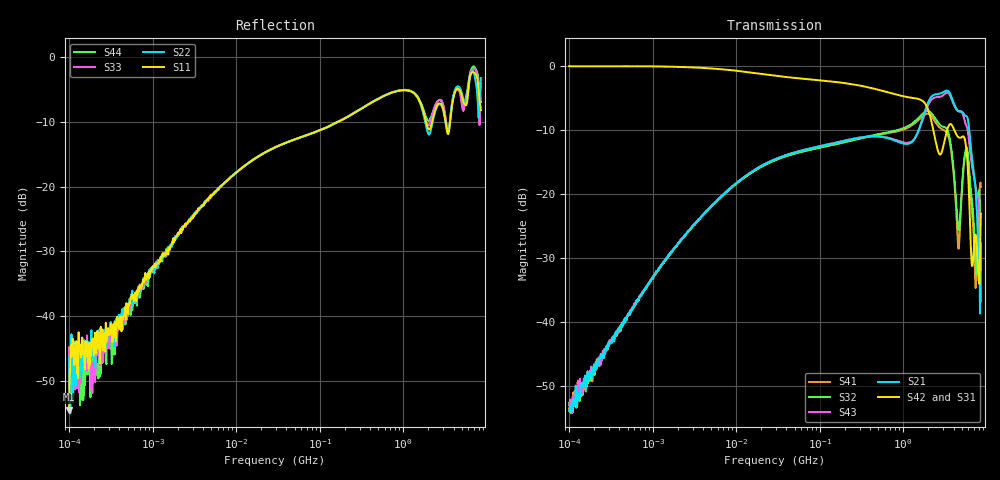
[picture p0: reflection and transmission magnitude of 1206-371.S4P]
!Agilent Technologies,E5071C,MY46110495,A.10.06
!Date: Tue Jun 06 11:07:04 2017
!Data & Calibration Information:
!Freq	S11:SOLT4(ON)	S12:SOLT4(ON)	S13:SOLT4(ON)	S14:SOLT4(ON)
!	S21:SOLT4(ON)	S22:SOLT4(ON)	S23:SOLT4(ON)	S24:SOLT4(ON)
!	S31:SOLT4(ON)	S32:SOLT4(ON)	S33:SOLT4(ON)	S34:SOLT4(ON)
!	S41:SOLT4(ON)	S42:SOLT4(ON)	S43:SOLT4(ON)	S44:SOLT4(ON)
!PortZ  Port1:50+j0  Port2:50+j0  Port3:50+j0  Port4:50+j0
!Above PortZ is port z conversion or system Z0 setting when saving the data.
!When reading, reference impedance value at option line is always used.
# Hz S dB R 50
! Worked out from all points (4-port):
!   801 points, 100 kHz to 8.5 GHz, reference 50 ohm
!   strongest paths, dB at 100 kHz, 1.721 MHz, 29.51 MHz, 502.3 MHz, 8.5 GHz:
!     S42: 0.0, -0.1, -1.5, -3.7, -23.1
!     S31: -0.1, -0.1, -1.5, -3.7, -27.3
!     S21: -53.9, -29.0, -14.6, -11.0, -27.8
!     S43: -53.1, -28.8, -14.6, -11.0, -27.8
!     S32: -52.7, -29.0, -14.7, -10.7, -28.0
!     S41: -53.5, -28.9, -14.7, -10.8, -18.9
!   lowest |S11| = -54.4 dB at 100 kHz (marker M1), VSWR 1.00, Z = 50.2 + j0.105 ohm
!   |S11| at or under -10 dB: start of sweep to 166.2 MHz; 1.867 GHz to 2.221 GHz (354.1 MHz wide, 17.3 % of centre); 3.211 GHz to 3.64 GHz (429 MHz wide, 12.5 % of centre)
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100000  -54.36 33.3  -55.71 82.1  -0.05 0.1  -53.83 -91.9
        -53.93 79.1  -46.27 7.1  -54.93 -84.9  -0.06 0.1
        -0.06 0.1  -52.70 -91.7  -44.76 96.1  -53.06 92.1
        -53.53 -99.3  -0.04 -0.1  -53.09 97.8  -47.70 63.1
9370604  -18.19 49.6  -18.64 47.9  -0.71 -5.9  -18.79 -132.7
         -18.66 48.0  -18.13 49.1  -18.74 -132.7  -0.71 -5.8
         -0.72 -5.8  -18.78 -132.9  -18.18 49.4  -18.64 47.9
         -18.70 -132.8  -0.70 -5.8  -18.64 48.0  -18.11 49.7
1.14275e9  -5.21 38.5  -12.17 22.4  -4.87 -34.1  -9.64 133.1
           -12.19 22.4  -5.18 37.2  -9.37 131.9  -4.91 -33.1
           -4.88 -34.1  -9.39 132.1  -5.21 36.7  -12.05 19.0
           -9.63 133.2  -4.90 -33.1  -12.03 19.1  -5.13 39.1
2.337209e9  -8.82 103.7  -4.51 21.8  -10.33 -74.6  -8.46 57.1
            -4.51 21.9  -9.07 106.2  -7.90 55.2  -10.59 -71.9
            -10.34 -74.6  -7.92 55.3  -8.06 102.9  -5.01 17.9
            -8.46 57.1  -10.59 -71.9  -5.00 17.8  -7.93 98.7
4.31778e9  -5.05 -131.3  -6.68 -22.4  -10.71 -78.4  -22.87 -33.2
           -6.68 -22.3  -4.71 -130.1  -21.40 -30.7  -10.71 -73.2
           -10.72 -78.2  -21.44 -30.7  -5.19 -136.8  -6.79 -27.9
           -22.79 -33.2  -10.70 -73.2  -6.79 -27.9  -4.95 -129.2
6.738951e9  -2.37 14.7  -14.90 -70.5  -31.50 -173.4  -23.45 -39.5
            -14.87 -70.5  -2.24 10.4  -21.77 -44.2  -31.34 -123.3
            -31.48 -172.9  -21.74 -43.8  -2.10 13.8  -16.07 -66.2
            -23.45 -39.3  -31.28 -122.9  -16.04 -65.9  -1.58 15.1
8.5e9  -8.23 103.2  -27.76 52.9  -27.28 86.5  -18.94 39.8
       -27.79 53.0  -3.30 117.4  -28.05 74.6  -23.12 3.1
       -27.29 86.7  -28.00 74.8  -4.12 122.8  -27.78 36.4
       -18.92 40.2  -23.09 3.6  -27.76 36.5  -6.96 88.4
